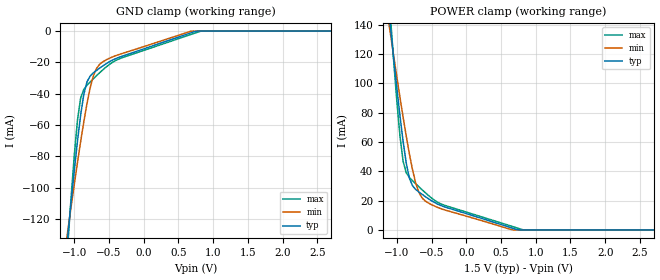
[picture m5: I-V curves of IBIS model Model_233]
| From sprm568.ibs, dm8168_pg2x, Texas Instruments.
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| Model based on original model for BSHTLTCSCDVGPBFZ
|   Sub model REC_FULLTERM_TH_1P5_6MA_10PER_1P5
[model]   Model_233
|[Description]  [1.5V-INPUT-FULLTERM:6MA-X, IND, 10%]
|   FULLTERM, 1.33 * RExt = 0.750 * Iout (I[2:0] = "001"), 6mA
|   nominal with Rext = 50R,Industrial temperature range (-40C to
|   125C, 25C nominal),10% power supply tolerance
|[Input Load]   FULLTERM:6MA
|[Output Drive]
|Voltage   1.5V
|Mode   INPUT
Model_type   Input
Polarity   Non-Inverting
Vinl =  0.65
Vinh =  1
C_comp   1.5249p   1.4275p   1.6205p
[Model Spec]
Vinl   0.65   0.65   0.65
Vinh   1   1   1
D_overshoot_high 1.95 1.95 1.95
D_overshoot_low -0.3 -0.3 -0.3
D_overshoot_time 1E-9 1E-9 1E-9
S_overshoot_high 1.65 1.65 1.65
S_overshoot_low 0 0 0
[Temperature Range]   25   125   -40
[Voltage Range]   1.5   1.35   1.65
[POWER_clamp]
-1.5V     337.1mA    270.3mA    433.1mA
-1.091V   138mA      133.4mA    144.8mA
-1.045V   117.1mA    118.8mA    115.4mA
-954.5mV  77.8mA     90.44mA    63.92mA
-909.1mV  60.19mA    76.83mA    46.76mA
-818.2mV  35.21mA    51.65mA    35.83mA
-727.3mV  27.61mA    31.83mA    31.51mA
-636.4mV  24.31mA    21.84mA    27.44mA
-545.5mV  21.36mA    18.41mA    23.61mA
-318.2mV  15.85mA    13.79mA    16.92mA
818.2mV   0A         0A         100.1uA
3V        0A         0A         0A
[GND_clamp]
-1.5V     -328.3mA   -263.1mA   -422.1mA
-1.091V   -129.4mA   -126.5mA   -134.5mA
-1.045V   -108.7mA   -112mA     -105.7mA
-954.5mV  -70.24mA   -83.95mA   -56.86mA
-909.1mV  -53.62mA   -70.61mA   -42.85mA
-863.6mV  -40.49mA   -57.99mA   -37.27mA
-818.2mV  -32.5mA    -46.42mA   -34.67mA
-727.3mV  -26.78mA   -28.82mA   -30.53mA
-590.9mV  -22.3mA    -19.68mA   -24.82mA
-363.6mV  -16.88mA   -15.09mA   -17.93mA
818.2mV   0A         0A         -103uA
3V        0A         0A         0A
